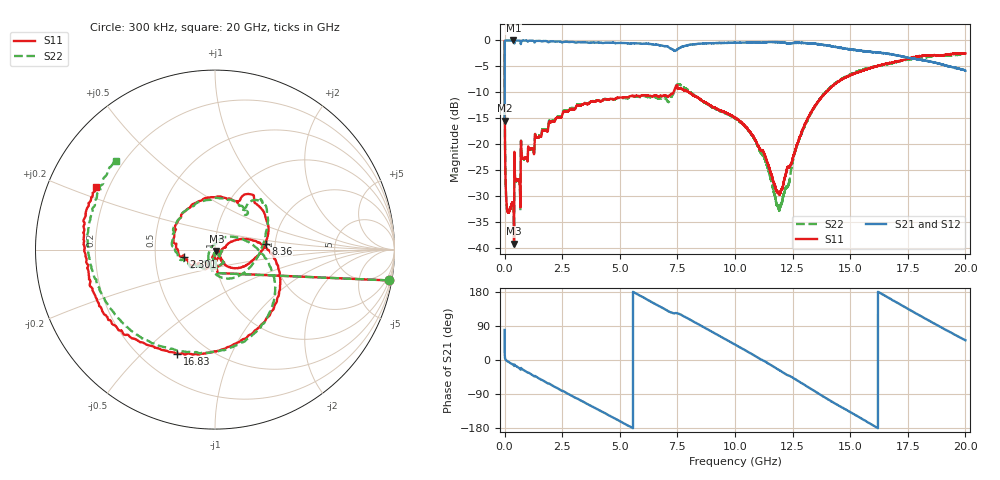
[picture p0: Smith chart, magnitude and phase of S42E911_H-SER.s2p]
! Created Wed Nov 25 22:29:11 2020
# khz S ma R 50
! 2 Port Network Data from SP1.SP block
! freq  magS11  angS11  magS21  angS21  magS12  angS12  magS22  angS22
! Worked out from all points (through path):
!   20001 points, 300 kHz to 20 GHz, reference 50 ohm
!   highest |S21| = 0.00 dB at 378.3 MHz (marker M1); lowest = -15.5 dB at 300 kHz (marker M2)
!   group delay of S21, straight-line fit = 93.2 ps
!   lowest |S11| = -39.1 dB at 410.3 MHz (marker M3), VSWR 1.02, Z = 50.7 - j0.845 ohm
!   |S11| at or under -10 dB: 5.272 MHz to 7.331 GHz (7.325 GHz wide, 200 % of centre); 8.005673 GHz to 8.007721 GHz (2.047 MHz wide, 0.0256 % of centre); 8.01 GHz to 13.95 GHz (5.94 GHz wide, 54.1 % of centre)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
!   |S22| runs from -39.6 to -0.1 dB; largest |S21 - S12| = 0.02
!   S11 on the Smith chart (normalised r, x): 300 kHz: 1, -11; 2.301 GHz: 0.70, -0.06; 8.36 GHz: 1.78, +0.12; 16.83 GHz: 0.34, -0.64; 20 GHz: 0.15, +0.24
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300  0.9851 -10.0  0.1684 79.4  0.1692 79.9  0.9837 -10.0
127300  0.02272 -96.2  0.9989 -3.5  0.9984 -3.5  0.02267 -96.0
378300  0.02614 -103.0  0.9996 -12.7  0.9986 -12.7  0.02569 -103.3
410300  0.01111 -48.6  0.9907 -15.0  0.99 -15.1  0.01047 -47.7
797300  0.07289 -114.7  0.9961 -25.6  0.9961 -25.6  0.07177 -117.0
2301300  0.1801 -166.4  0.9775 -74.8  0.9777 -74.8  0.1841 -161.8
3334300  0.2387 161.3  0.9603 -107.8  0.9595 -107.8  0.243 165.9
5123300  0.2825 110.5  0.9448 -165.3  0.944 -165.4  0.2789 102.5
6667300  0.2902 70.7  0.9066 143.3  0.9058 143.2  0.2748 54.5
7430300  0.3593 59.6  0.7978 123.9  0.7977 124.0  0.3615 49.7
8360300  0.2837 6.2  0.9255 96.2  0.9219 96.3  0.2854 12.4
9169300  0.222 -14.7  0.9445 68.8  0.9469 68.8  0.219 -26.3
1.00003e7  0.1811 -32.4  0.9498 40.7  0.9507 40.8  0.1781 -65.1
1.12503e7  0.08295 -58.8  0.9561 -2.1  0.9552 -2.1  0.07565 -115.7
1.19083e7  0.03384 -20.6  0.9639 -26.3  0.9643 -26.3  0.02337 143.4
1.33343e7  0.2079 15.2  0.9335 -77.7  0.9325 -77.5  0.206 8.6
1.41373e7  0.3489 -12.1  0.8858 -107.5  0.8855 -107.1  0.3537 -23.5
1.51543e7  0.4761 -50.9  0.8085 -142.8  0.8162 -143.1  0.4873 -55.4
1.66673e7  0.5993 -104.7  0.7427 164.3  0.7275 164.2  0.5937 -107.4
1.68303e7  0.6161 -110.0  0.7318 158.2  0.7151 158.5  0.6044 -113.8
1.84383e7  0.7149 -157.1  0.6278 103.2  0.6284 103.8  0.6982 -173.4
2e7  0.7504 152.1  0.5124 52.0  0.514 53.1  0.7393 138.0
